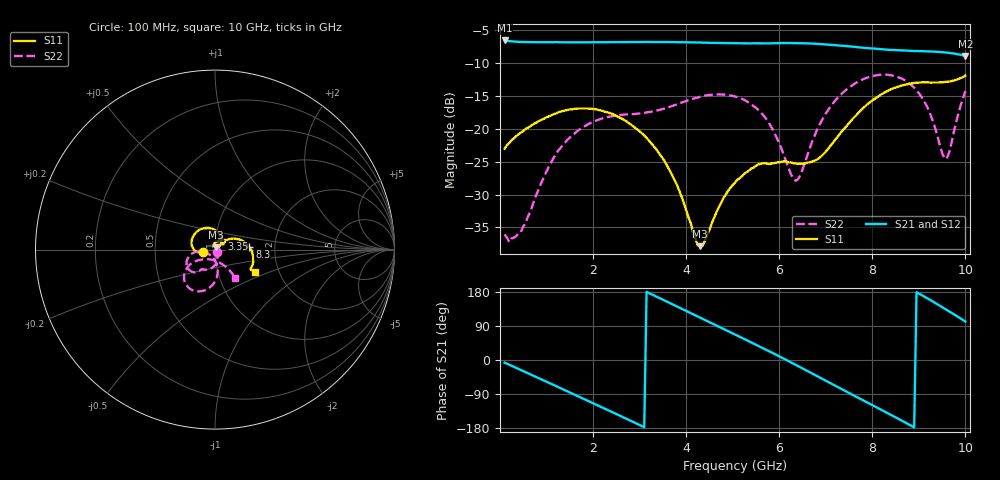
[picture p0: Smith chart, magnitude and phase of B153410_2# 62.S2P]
!  2-Port S-parameters saved by WinCal
! VAR MeasName=S-Parameters (CALIBRATED_DATA) read from VNA (N5245A)
! VAR MeasDate=2016-12-23 10:02:42
! VAR NAME=B153410_2# 62
! VAR FILENAME=B153410_2# 62.S2P
! VAR DATE=2016-12-23 10:02:42
! VAR PHYS_PORTS=1,2
# Hz S DB R 50
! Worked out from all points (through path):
!   199 points, 100 MHz to 10 GHz, reference 50 ohm
!   highest |S21| = -6.54 dB at 100 MHz (marker M1); lowest = -8.9 dB at 10 GHz (marker M2)
!   group delay of S21, straight-line fit = 170 ps
!   lowest |S11| = -37.9 dB at 4.3 GHz (marker M3), VSWR 1.03, Z = 50.4 + j1.22 ohm
!   |S11| at or under -10 dB: start of sweep to end of sweep
!   |S22| runs from -37.2 to -11.7 dB; largest |S21 - S12| = 0.0036
!   S11 on the Smith chart (normalised r, x): 100 MHz: 0.87, -0.02; 3.35 GHz: 1.07, +0.13; 8.3 GHz: 1.47, +0.04; 10 GHz: 1.51, -0.40
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1e8  -23.01 -169.9  -6.54 -6.9  -6.55 -6.9  -36.06 -53.3
2e8  -22.15 -168.6  -6.65 -12.5  -6.64 -12.5  -37.23 -75.2
4.5e8  -20.59 -170.8  -6.77 -26.4  -6.76 -26.4  -35.70 -78.6
1.2e9  -17.66 169.7  -6.80 -68.5  -6.80 -68.6  -23.82 -78.7
1.75e9  -16.89 145.2  -6.83 -99.7  -6.83 -99.8  -19.89 -98.7
2.65e9  -18.56 97.8  -6.78 -151.2  -6.81 -151.2  -17.85 -120.7
3.35e9  -23.03 58.9  -6.78 168.0  -6.78 168.0  -17.24 -124.9
3.4e9  -23.53 56.2  -6.79 165.0  -6.79 165.1  -17.15 -124.8
3.8e9  -28.49 39.1  -6.81 141.4  -6.81 141.5  -16.28 -126.8
4.3e9  -37.86 70.8  -6.85 111.8  -6.86 111.8  -15.12 -134.4
5.05e9  -28.19 90.9  -6.97 67.2  -6.97 67.3  -15.06 -153.9
5.75e9  -25.32 50.9  -6.99 25.1  -7.00 25.3  -18.79 -172.8
6.35e9  -25.25 32.2  -6.94 -12.6  -6.97 -12.4  -27.90 -131.2
6.7e9  -24.99 33.7  -7.01 -35.1  -7.03 -35.0  -22.07 -83.8
7.35e9  -20.34 37.1  -7.35 -77.2  -7.36 -77.2  -14.60 -91.7
7.8e9  -16.84 23.7  -7.65 -106.3  -7.67 -105.9  -12.44 -106.0
8.3e9  -14.32 4.1  -7.93 -138.3  -7.95 -137.9  -11.75 -123.3
8.35e9  -14.15 2.2  -7.96 -141.5  -7.97 -141.2  -11.78 -125.1
9.05e9  -12.93 -21.5  -8.16 172.1  -8.16 172.4  -15.07 -147.9
9.55e9  -12.87 -29.1  -8.36 136.0  -8.36 136.3  -24.47 -111.6
9.65e9  -12.80 -29.2  -8.43 128.5  -8.43 128.8  -23.63 -80.4
1e10  -11.89 -29.1  -8.92 101.6  -8.92 101.9  -14.24 -54.5
